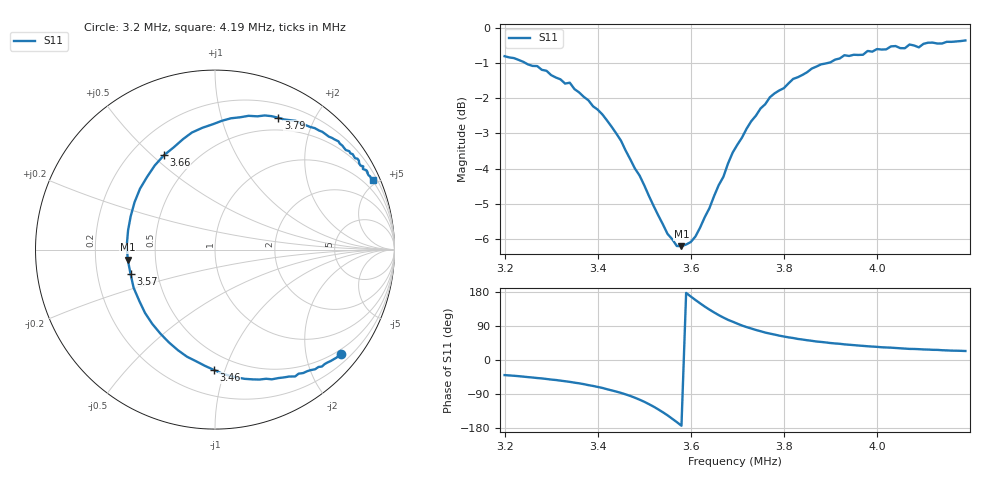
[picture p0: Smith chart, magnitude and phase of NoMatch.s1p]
! Touchstone file generated by AntScope (RigExpert AA-54 antenna analyzer)
# MHz Z RI R 50
! Format: Frequency Z-real Z-imaginary (normalized to 50 Ohm)
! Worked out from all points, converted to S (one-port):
!   100 points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, 3.2 MHz to 4.19 MHz, reference 50 ohm
!   lowest |S11| = -6.2 dB at 3.58 MHz (marker M1), VSWR 2.92, Z = 17.2 - j2.52 ohm
!   |S11| at or under -10 dB: nowhere
!   S11 on the Smith chart (normalised r, x): 3.2 MHz: 0.39, -2.71; 3.46 MHz: 0.38, -0.91; 3.57 MHz: 0.35, -0.12; 3.66 MHz: 0.33, +0.55; 3.79 MHz: 0.35, +1.53; 4.19 MHz: 0.48, +4.71
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3.2  0.3912 -2.708
3.27  0.3756 -2.216
3.33  0.3998 -1.811
3.36  0.3896 -1.612
3.4  0.3802 -1.329
3.45  0.3726 -0.9858
3.46  0.3768 -0.9144
3.49  0.366 -0.705
3.52  0.3584 -0.4884
3.54  0.3518 -0.3428
3.57  0.3486 -0.1246
3.58  0.3438 -0.0504
3.6  0.3404 0.0972
3.62  0.3366 0.243
3.64  0.3356 0.392
3.66  0.3336 0.5454
3.68  0.3334 0.699
3.7  0.3328 0.8448
3.73  0.3346 1.072
3.75  0.3366 1.225
3.79  0.3508 1.534
3.82  0.3464 1.753
3.87  0.3628 2.155
3.93  0.3538 2.614
3.95  0.3822 2.755
4.07  0.4184 3.784
4.09  0.513 3.863
4.19  0.4774 4.708
